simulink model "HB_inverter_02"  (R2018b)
settings: Solver=VariableStepAuto  StartTime=0.0  StopTime=0.02  MaxStep=1e-6  RelTol=1e-7
libraries: powerlib x6, simulink x1

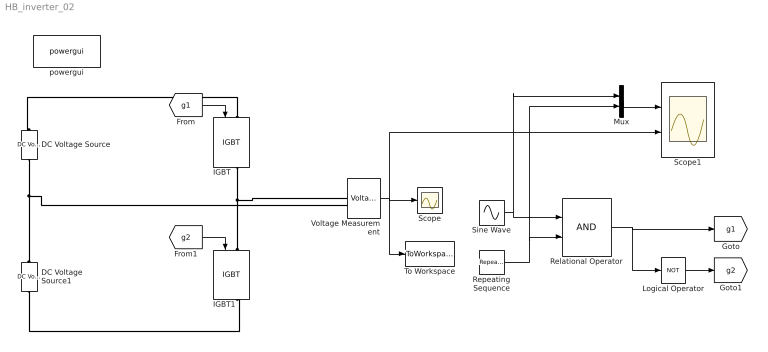
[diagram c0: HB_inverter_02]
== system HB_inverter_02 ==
  DC Voltage Source : powerlib/Electrical Sources/DC Voltage Source  Amplitude=100  Measurements=None
  DC Voltage Source1 : powerlib/Electrical Sources/DC Voltage Source  Amplitude=100  Measurements=None
  IGBT : powerlib/Power Electronics/IGBT  Ron=0.001  Lon=0  Vf=1  Tf=1e-6  Tt=2e-6  IC=0  Rs=1e5  Cs=inf  Measurements=on
  IGBT1 : powerlib/Power Electronics/IGBT  Ron=0.001  Lon=0  Vf=1  Tf=1e-6  Tt=2e-6  IC=0  Rs=1e5  Cs=inf  Measurements=on
  Logical Operator : Logic  Operator=NOT  AllPortsSameDT=off  OutDataTypeStr=boolean
  Mux : Mux  Inputs=2
  Relational Operator : RelationalOperator  OutDataTypeStr=boolean  RndMeth=Simplest
  Repeating Sequence : simulink/Sources/Repeating Sequence  rep_seq_t=[0 0.00005 0.0001]  rep_seq_y=[-100 100 -100]
  Scope : Scope
  Scope1 : Scope  NumInputPorts=2
  Sine Wave : Sin  Amplitude=90  Frequency=2*pi*100  SampleTime=0
  To Workspace : ToWorkspace  VariableName=vo  SaveFormat=Structure With Time  SampleTime=-1
  Voltage Measurement : powerlib/Measurements/Voltage Measurement  PhasorSimulation=off  OutputType=Complex  PSBequivalent=0
  powergui : powerlib/powergui  Priority=1  SimulationMode=Continuous  SampleTime=50e-6  frequency=60  Iterations=50  frequencyindice=0  Pbase=100e6  ErrMax=1e-4  UnitsV=kV  UnitsW=MW  buscounter=0  FunctionMessages=on  echomessages=on  EnableUseOfTLC=off  CurrentSourceSwitches=off  DisableSnubberDevices=off  DisableRonSwitches=off  DisableVfSwitches=off  DisplayEquations=off  SolverType=Tustin/Backward Euler (TBE)  Interpol=off  ExternalGateDelay=off  methode=off  Ts=100  x0status=blocks  SPID=on  SwTol=0  HookPort=off  RestoreLinks=warning  ResistiveCurrentMeasurement=off  Frange=[0:2:500]  Ylog=off  Xlog=on  ShowGrid=off  save=off  variable=ZData  structure=vo  ZoomFFT=off  StartTime=0.0  cycles=1  DisplayStyle=1  fundamental=100  FreqAxis=off  MaxFrequency=100000  frequencyindicesteady=1  RmsSteady=1  display=off
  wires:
  [g1] -> IGBT/1
  [g2] -> IGBT1/1
  Repeating Sequence/1 -> Mux/2, Relational Operator/2
  Sine Wave/1 -> Mux/1, Relational Operator/1
  Relational Operator/1 -> Logical Operator/1, [g1]
  Logical Operator/1 -> [g2]
  Mux/1 -> Scope1/1
  Voltage Measurement/1 -> Scope1/2, To Workspace/1, Scope/1
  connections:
  IGBT1/LConn1 -- Voltage Measurement/LConn1 -- IGBT/RConn1
  IGBT/LConn1 -- DC Voltage Source/RConn1
  DC Voltage Source1/LConn1 -- IGBT1/RConn1
  DC Voltage Source/LConn1 -- Voltage Measurement/LConn2 -- DC Voltage Source1/RConn1
